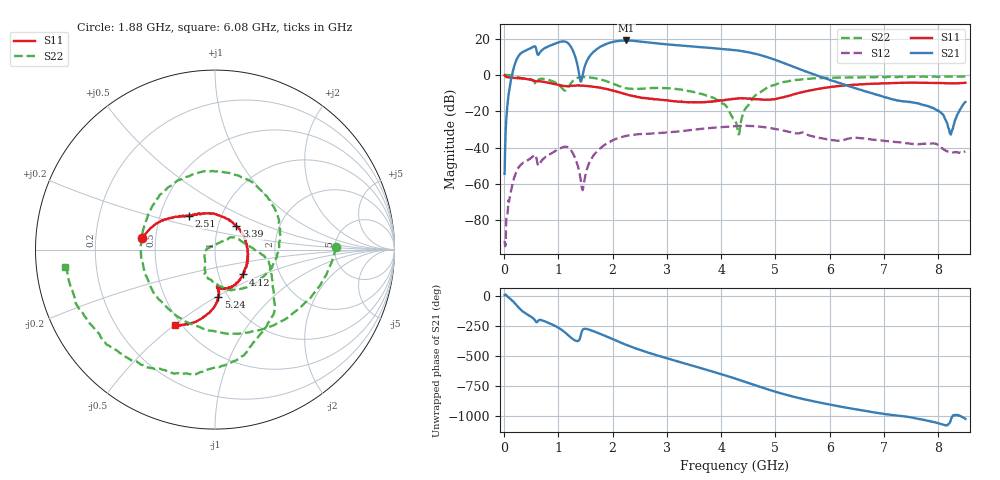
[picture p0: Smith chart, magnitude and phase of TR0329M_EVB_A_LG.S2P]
!Agilent Technologies,E5071C,MY46523237,B.13.01
!Date: Thu Mar 10 13:18:05 2022
!Data & Calibration Information:
!Freq	S11:SOLT2(ON)	S21:SOLT2(ON)	S12:SOLT2(ON)	S22:SOLT2(ON)
!PortZ  Port1:50+j0  Port2:50+j0
!Above PortZ is port z conversion or system Z0 setting when saving the data.
!When reading, reference impedance value at option line is always used.
# Hz S dB R 50
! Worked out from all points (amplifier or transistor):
!   850 points, 10 MHz to 8.5 GHz, reference 50 ohm
!   highest |S21| = 18.9 dB at 2.25 GHz (marker M1)
!   |S21| within 3 dB of that: 1.807 GHz to 3.336 GHz (1.529 GHz wide, 59.5 % of centre)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
!   unconditionally stable (mu >= 1): 12.53 MHz to end of sweep
!   at 1.42 GHz: K = 130.98, MAG = 3.7 dB, |S12| = -59.3 dB
!   at 4.26 GHz: K = 2.63, MAG = 13.8 dB, |S12| = -28.1 dB
!   at 8.5 GHz: K = 43.76, MAG = -5.7 dB, |S12| = -42.3 dB
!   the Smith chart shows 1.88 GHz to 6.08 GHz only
!   S11 on the Smith chart (normalised r, x): 1.88 GHz: 0.42, +0.06; 2.51 GHz: 0.70, +0.28; 3.39 GHz: 1.22, +0.33; 4.12 GHz: 1.31, -0.38; 5.24 GHz: 0.90, -0.51; 6.08 GHz: 0.46, -0.51
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1e7  -0.26 -4.5  -54.40 7.2  -91.24 134.4  0.01 -72.8
3.1e8  -1.87 -40.6  11.86 -115.5  -49.34 88.1  -1.71 147.8
5.3e8  -2.97 -68.3  15.31 176.6  -44.86 38.1  -2.91 121.7
8.7e8  -4.64 -101.3  16.34 125.6  -43.12 9.8  -3.21 78.2
1.04e9  -5.77 -115.0  18.24 84.6  -40.35 -21.3  -6.36 17.1
1.2e9  -6.20 -123.1  16.79 25.8  -40.12 -76.6  -6.02 -131.4
1.3e9  -5.84 -130.9  10.99 -8.5  -45.10 -114.3  -2.48 163.9
1.43e9  -5.88 -144.4  -2.58 61.1  -61.90 172.6  -1.27 114.9
1.68e9  -6.63 -169.5  13.49 60.6  -43.15 9.2  -1.85 51.4
1.88e9  -7.68 171.1  16.96 23.7  -37.95 -24.2  -3.41 1.4
2.25e9  -10.71 141.9  18.93 -46.6  -33.51 -85.6  -7.37 -115.8
2.51e9  -12.41 128.0  18.32 -90.7  -32.54 -123.7  -7.65 166.5
2.84e9  -13.51 106.1  17.24 -137.6  -32.03 -164.0  -7.11 98.5
3.39e9  -15.04 47.8  15.83 150.1  -30.53 133.8  -8.91 5.9
4.12e9  -13.64 -41.7  13.97 52.3  -28.52 41.1  -18.19 -118.3
4.26e9  -13.02 -54.8  13.53 32.3  -28.14 22.2  -25.16 -173.7
4.74e9  -13.51 -86.5  10.74 -40.0  -28.54 -48.5  -9.17 -24.6
5.24e9  -11.58 -85.9  5.58 -107.9  -31.25 -113.6  -3.50 -93.2
5.67e9  -8.38 -99.9  0.65 -153.8  -33.67 -161.9  -1.99 -137.1
6.08e9  -6.44 -117.5  -3.48 169.6  -35.96 168.5  -1.53 -173.5
7.09e9  -4.57 -163.7  -12.81 92.9  -36.42 66.5  -1.03 92.8
8.5e9  -4.36 110.1  -14.90 56.4  -42.28 -89.6  -0.91 -20.8
